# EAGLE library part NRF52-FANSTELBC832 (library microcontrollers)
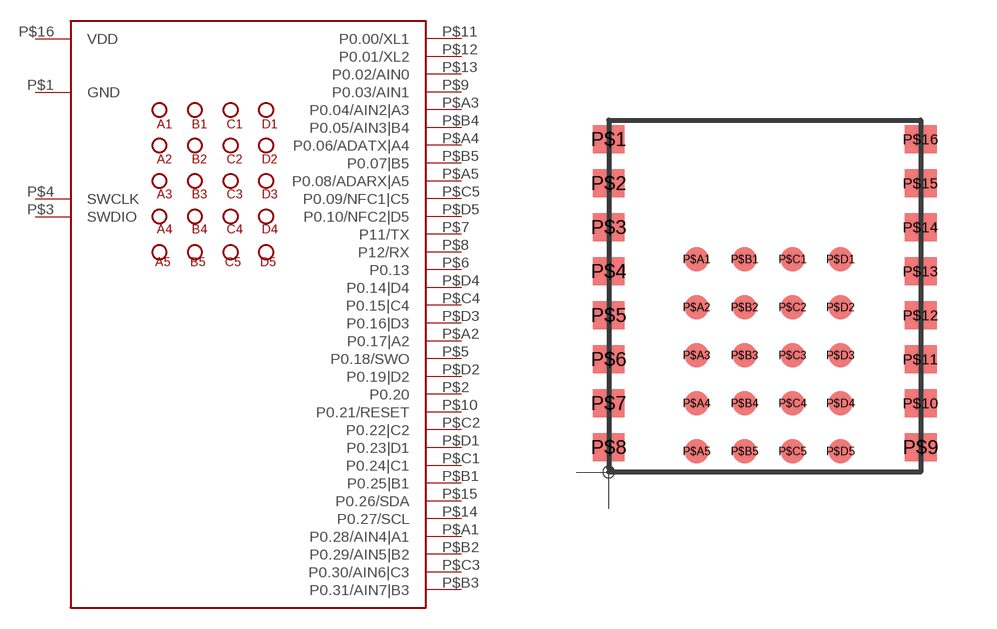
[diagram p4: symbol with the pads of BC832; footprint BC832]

Designator prefix U

## NRF52-FANSTELBC832  [BC832]
P$1  GND
P$2  P0.20
P$3  SWDIO
P$4  SWCLK
P$5  P0.18/SWO
P$6  P0.13
P$7  P11/TX
P$8  P12/RX
P$9  P0.03/AIN1
P$10  P0.21/RESET
P$11  P0.00/XL1
P$12  P0.01/XL2
P$13  P0.02/AIN0
P$14  P0.27/SCL
P$15  P0.26/SDA
P$16  VDD
P$A1  P0.28/AIN4|A1
P$A2  P0.17|A2
P$A3  P0.04/AIN2|A3
P$A4  P0.06/ADATX|A4
P$A5  P0.08/ADARX|A5
P$B1  P0.25|B1
P$B2  P0.29/AIN5|B2
P$B3  P0.31/AIN7|B3
P$B4  P0.05/AIN3|B4
P$B5  P0.07|B5
P$C1  P0.24|C1
P$C2  P0.22|C2
P$C3  P0.30/AIN6|C3
P$C4  P0.15|C4
P$C5  P0.09/NFC1|C5
P$D1  P0.23|D1
P$D2  P0.19|D2
P$D3  P0.16|D3
P$D4  P0.14|D4
P$D5  P0.10/NFC2|D5

## Footprint BC832 (pad centres in mm)
smd 0.8 x 0.7: P$1 0,8.32; P$2 0,7.22; P$3 0,6.12; P$4 0,5.02; P$5 0,3.92; P$6 0,2.82; P$7 0,1.72; P$8 0,0.62; P$9 7.8,0.62; P$10 7.8,1.72; P$11 7.8,2.82; P$12 7.8,3.92; P$13 7.8,5.02; P$14 7.8,6.12; P$15 7.8,7.22; P$16 7.8,8.32
smd 0.6 x 0.6: P$A1 2.2,5.319; P$A2 2.2,4.119; P$A3 2.2,2.919; P$A4 2.2,1.719; P$A5 2.2,0.519; P$B1 3.4,5.319; P$B2 3.4,4.119; P$B3 3.4,2.919; P$B4 3.4,1.719; P$B5 3.4,0.519; P$C1 4.6,5.319; P$C2 4.6,4.119; P$C3 4.6,2.919; P$C4 4.6,1.719; P$C5 4.6,0.519; P$D1 5.8,5.319; P$D2 5.8,4.119; P$D3 5.8,2.919; P$D4 5.8,1.719; P$D5 5.8,0.519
